| Teraspeed Labs Modeling Services.
| http://www.teraspeedlabs.com
[IBIS Ver]  4.0
[File Name] ev12ds400azpy-v2.ibs
[File Rev]  3.1
[Source]  Created by Teraspeed Labs LLC
[Date]   05/12/2015
[Notes]   Quality Check of this IBIS model: Model Passes IBIS Check
   Model parses into ICX IS. Simulation done with Hyperlynx.
   1. MIN TYP MAX information is based on Temperature and
   Voltage characteristics only.
   2. Package data gained using Tektronix IConnect Software.
   3. File Rev3.1: changed ball F10 from DGND to VCCD(from PDF)
[Disclaimer]
| Use: Teraspeed Labs  ("Teraspeed") has
| licensed IBIS models to specific integrated circuit
| suppliers ("IC Vendors") for use and distribution as
| follows: Each IC Vendor may use IBIS Models, and distribute
| them to IC Vendor's customers to use solely for developing
| printed circuit board designs. Users of this model may
| modify the IBIS model to suit its specific applications but
| rights to derivative works and such modifications shall belong
| to Teraspeed. No other distribution of these materials is
| permitted.
| DISCLAIMER OF WARRANTY: UNLESS OTHERWISE AGREED TO IN WRITING
| TERASPEED DISCLAIMS AND USER WAIVES ALL WARRANTIES, EXPRESS
| OR IMPLIED, INCLUDING WARRANTIES OF MERCHANTABILITY AND
| FITNESS FOR A PARTICULAR PURPOSE. IN NO EVENT SHALL
| TERASPEED BE LIABLE FOR ANY DIRECT OR INDIRECT DAMAGES,
| WHETHER IN CONTRACT OR TORT, INCLUDING, WITHOUT LIMITATION,
| LOST PROFITS, BUSINESS INTERRUPTION, OR LOST INFORMATION
| ARISING OUT OF THE USE OF OR THE INABILITY TO USE THE MODEL,
| EVEN IF TERASPEED HAS BEEN ADVISED OF THE POSSIBILITY OF SUCH
| DAMAGES.
[Copyright]
| This file is the legal property of Teraspeed Labs Copyright(c) 2015.
| All other rights are reserved.
[Component]   EV12DS400AZPY-v2
[Manufacturer] e2v semiconductors
| Data Sheet: Preliminary - SEPT 14/Extract of Product Brief
[Package]
| FpBGA196 ROHS
| variable   typ   min   max
R_pkg  1.000E-02   1.000E-02   1.000E-02
L_pkg  1.293E-09   1.711E-10   2.224E-09
C_pkg  4.897E-13   6.478E-14   8.421E-13
[Pin] signal_name   model_name   R_pin   L_pin   C_pin
A1   DGND   GND   1.000E-02   2.224E-09   8.421E-13
A2   B5   lvds_in   1.000E-02   2.060E-09   7.800E-13
A3   B6   lvds_in   1.000E-02   1.913E-09   7.242E-13
A4   B6N   lvds_in   1.000E-02   1.786E-09   6.763E-13
A5   B9   lvds_in   1.000E-02   1.685E-09   6.380E-13
A6   B9N   lvds_in   1.000E-02   1.614E-09   6.111E-13
A7   B11   lvds_in   1.000E-02   1.577E-09   5.972E-13
A8   C11   lvds_in   1.000E-02   1.577E-09   5.972E-13
A9   C9N   lvds_in   1.000E-02   1.614E-09   6.111E-13
A10   C9   lvds_in   1.000E-02   1.685E-09   6.380E-13
A11   C6N   lvds_in   1.000E-02   1.786E-09   6.763E-13
A12   C6   lvds_in   1.000E-02   1.913E-09   7.242E-13
A13   C5   lvds_in   1.000E-02   2.060E-09   7.800E-13
A14   DGND   GND   1.000E-02   2.224E-09   8.421E-13
B1   B3   lvds_in   1.000E-02   2.060E-09   7.800E-13
B2   B4   lvds_in   1.000E-02   1.882E-09   7.125E-13
B3   B5N   lvds_in   1.000E-02   1.719E-09   6.510E-13
B4   B7   lvds_in   1.000E-02   1.577E-09   5.972E-13
B5   B8   lvds_in   1.000E-02   1.462E-09   5.534E-13
B6   B10   lvds_in   1.000E-02   1.379E-09   5.222E-13
B7   B11N   lvds_in   1.000E-02   1.336E-09   5.059E-13
B8   C11N   lvds_in   1.000E-02   1.336E-09   5.059E-13
B9   C10   lvds_in   1.000E-02   1.379E-09   5.222E-13
B10   C8   lvds_in   1.000E-02   1.462E-09   5.534E-13
B11   C7   lvds_in   1.000E-02   1.577E-09   5.972E-13
B12   C5N   lvds_in   1.000E-02   1.719E-09   6.510E-13
B13   C4   lvds_in   1.000E-02   1.882E-09   7.125E-13
B14   C3   lvds_in   1.000E-02   2.060E-09   7.800E-13
C1   B1N   lvds_in   1.000E-02   1.913E-09   7.242E-13
C2   B3N   lvds_in   1.000E-02   1.719E-09   6.510E-13
C3   B4N   lvds_in   1.000E-02   1.540E-09   5.830E-13
C4   B7N   lvds_in   1.000E-02   1.379E-09   5.222E-13
C5   B8N   lvds_in   1.000E-02   1.245E-09   4.716E-13
C6   B10N   lvds_in   1.000E-02   1.148E-09   4.345E-13
C7   DGND   GND   1.000E-02   1.095E-09   4.148E-13
C8   DGND   GND   1.000E-02   1.095E-09   4.148E-13
C9   C10N   lvds_in   1.000E-02   1.148E-09   4.345E-13
C10   C8N   lvds_in   1.000E-02   1.245E-09   4.716E-13
C11   C7N   lvds_in   1.000E-02   1.379E-09   5.222E-13
C12   C4N   lvds_in   1.000E-02   1.540E-09   5.830E-13
C13   C3N   lvds_in   1.000E-02   1.719E-09   6.510E-13
C14   C1N   lvds_in   1.000E-02   1.913E-09   7.242E-13
D1   B1   lvds_in   1.000E-02   1.786E-09   6.763E-13
D2   B2   lvds_in   1.000E-02   1.577E-09   5.972E-13
D3   B2N   lvds_in   1.000E-02   1.379E-09   5.222E-13
D4   DGND   GND   1.000E-02   1.198E-09   4.534E-13
D5   DGND   GND   1.000E-02   1.041E-09   3.940E-13
D6   VCCD   POWER   1.000E-02   9.213E-10   3.488E-13
D7   VCCD   POWER   1.000E-02   8.554E-10   3.239E-13
D8   VCCD   POWER   1.000E-02   8.554E-10   3.239E-13
D9   VCCD   POWER   1.000E-02   9.213E-10   3.488E-13
D10   DGND   GND   1.000E-02   1.041E-09   3.940E-13
D11   DGND   GND   1.000E-02   1.198E-09   4.534E-13
D12   C2N   lvds_in   1.000E-02   1.379E-09   5.222E-13
D13   C2   lvds_in   1.000E-02   1.577E-09   5.972E-13
D14   C1   lvds_in   1.000E-02   1.786E-09   6.763E-13
E1   A10N   lvds_in   1.000E-02   1.685E-09   6.380E-13
E2   B0   lvds_in   1.000E-02   1.462E-09   5.534E-13
E3   B0N   lvds_in   1.000E-02   1.245E-09   4.716E-13
E4   DGND   GND   1.000E-02   1.041E-09   3.940E-13
E5   DGND   GND   1.000E-02   8.554E-10   3.239E-13
E6   VCCD   POWER   1.000E-02   7.054E-10   2.671E-13
E7   VCCD   POWER   1.000E-02   6.168E-10   2.336E-13
E8   VCCD   POWER   1.000E-02   6.168E-10   2.336E-13
E9   VCCD   POWER   1.000E-02   7.054E-10   2.671E-13
E10   DGND   GND   1.000E-02   8.554E-10   3.239E-13
E11   DGND   GND   1.000E-02   1.041E-09   3.940E-13
E12   C0N   lvds_in   1.000E-02   1.245E-09   4.716E-13
E13   C0   lvds_in   1.000E-02   1.462E-09   5.534E-13
E14   D10N   lvds_in   1.000E-02   1.685E-09   6.380E-13
F1   A10   lvds_in   1.000E-02   1.614E-09   6.111E-13
F2   A11   lvds_in   1.000E-02   1.379E-09   5.222E-13
F3   A11N   lvds_in   1.000E-02   1.148E-09   4.345E-13
F4   VCCD   POWER   1.000E-02   9.213E-10   3.488E-13
F5   VCCD   POWER   1.000E-02   7.054E-10   2.671E-13
F6   AGND   GND   1.000E-02   5.132E-10   1.943E-13
F7   AGND   GND   1.000E-02   3.825E-10   1.448E-13
F8   AGND   GND   1.000E-02   3.825E-10   1.448E-13
F9   AGND   GND   1.000E-02   5.132E-10   1.943E-13
F10   VCCD   POWER   1.000E-02   7.054E-10   2.671E-13
F11   VCCD   POWER   1.000E-02   9.213E-10   3.488E-13
F12   D11N   lvds_in   1.000E-02   1.148E-09   4.345E-13
F13   D11   lvds_in   1.000E-02   1.379E-09   5.222E-13
F14   D10   lvds_in   1.000E-02   1.614E-09   6.111E-13
G1   A8   lvds_in   1.000E-02   1.577E-09   5.972E-13
G2   A8N   lvds_in   1.000E-02   1.336E-09   5.059E-13
G3   A9   lvds_in   1.000E-02   1.095E-09   4.148E-13
G4   A9N   lvds_in   1.000E-02   8.554E-10   3.239E-13
G5   DGND   GND   1.000E-02   6.168E-10   2.336E-13
G6   AGND   GND   1.000E-02   3.825E-10   1.448E-13
G7   AGND   GND   1.000E-02   1.711E-10   6.478E-14
G8   AGND   GND   1.000E-02   1.711E-10   6.478E-14
G9   AGND   GND   1.000E-02   3.825E-10   1.448E-13
G10   DGND   GND   1.000E-02   6.168E-10   2.336E-13
G11   D9N   lvds_in   1.000E-02   8.554E-10   3.239E-13
G12   D9   lvds_in   1.000E-02   1.095E-09   4.148E-13
G13   D8N   lvds_in   1.000E-02   1.336E-09   5.059E-13
G14   D8   lvds_in   1.000E-02   1.577E-09   5.972E-13
H1   A6   lvds_in   1.000E-02   1.577E-09   5.972E-13
H2   A6N   lvds_in   1.000E-02   1.336E-09   5.059E-13
H3   A7   lvds_in   1.000E-02   1.095E-09   4.148E-13
H4   A7N   lvds_in   1.000E-02   8.554E-10   3.239E-13
H5   DGND   GND   1.000E-02   6.168E-10   2.336E-13
H6   AGND   GND   1.000E-02   3.825E-10   1.448E-13
H7   AGND   GND   1.000E-02   1.711E-10   6.478E-14
H8   AGND   GND   1.000E-02   1.711E-10   6.478E-14
H9   AGND   GND   1.000E-02   3.825E-10   1.448E-13
H10   DGND   GND   1.000E-02   6.168E-10   2.336E-13
H11   D7N   lvds_in   1.000E-02   8.554E-10   3.239E-13
H12   D7   lvds_in   1.000E-02   1.095E-09   4.148E-13
H13   D6N   lvds_in   1.000E-02   1.336E-09   5.059E-13
H14   D6   lvds_in   1.000E-02   1.577E-09   5.972E-13
J1   A3N   lvds_in   1.000E-02   1.614E-09   6.111E-13
J2   A5   lvds_in   1.000E-02   1.379E-09   5.222E-13
J3   A5N   lvds_in   1.000E-02   1.148E-09   4.345E-13
J4   VCCA3   POWER   1.000E-02   9.213E-10   3.488E-13
J5   VCCA3   POWER   1.000E-02   7.054E-10   2.671E-13
J6   AGND   GND   1.000E-02   5.132E-10   1.943E-13
J7   AGND   GND   1.000E-02   3.825E-10   1.448E-13
J8   AGND   GND   1.000E-02   3.825E-10   1.448E-13
J9   AGND   GND   1.000E-02   5.132E-10   1.943E-13
J10   VCCA3   POWER   1.000E-02   7.054E-10   2.671E-13
J11   VCCA3   POWER   1.000E-02   9.213E-10   3.488E-13
J12   D5N   lvds_in   1.000E-02   1.148E-09   4.345E-13
J13   D5   lvds_in   1.000E-02   1.379E-09   5.222E-13
J14   D3N   lvds_in   1.000E-02   1.614E-09   6.111E-13
K1   A3   lvds_in   1.000E-02   1.685E-09   6.380E-13
K2   A4   lvds_in   1.000E-02   1.462E-09   5.534E-13
K3   A4N   lvds_in   1.000E-02   1.245E-09   4.716E-13
K4   DGND   GND   1.000E-02   1.041E-09   3.940E-13
K5   DGND   GND   1.000E-02   8.554E-10   3.239E-13
K6   AGND   GND   1.000E-02   7.054E-10   2.671E-13
K7   VCCA5   POWER   1.000E-02   6.168E-10   2.336E-13
K8   VCCA5   POWER   1.000E-02   6.168E-10   2.336E-13
K9   AGND   GND   1.000E-02   7.054E-10   2.671E-13
K10   DGND   GND   1.000E-02   8.554E-10   3.239E-13
K11   DGND   GND   1.000E-02   1.041E-09   3.940E-13
K12   D4N   lvds_in   1.000E-02   1.245E-09   4.716E-13
K13   D4   lvds_in   1.000E-02   1.462E-09   5.534E-13
K14   D3   lvds_in   1.000E-02   1.685E-09   6.380E-13
L1   A1N   lvds_in   1.000E-02   1.786E-09   6.763E-13
L2   A2   lvds_in   1.000E-02   1.577E-09   5.972E-13
L3   A2N   lvds_in   1.000E-02   1.379E-09   5.222E-13
L4   DGND   GND   1.000E-02   1.198E-09   4.534E-13
L5   DIODE   term   1.000E-02   1.041E-09   3.940E-13
L6   VCCA5   POWER   1.000E-02   9.213E-10   3.488E-13
L7   VCCA5   POWER   1.000E-02   8.554E-10   3.239E-13
L8   VCCA5   POWER   1.000E-02   8.554E-10   3.239E-13
L9   VCCA5   POWER   1.000E-02   9.213E-10   3.488E-13
L10   DGND   GND   1.000E-02   1.041E-09   3.940E-13
L11   SLD_N   spi_in   1.000E-02   1.198E-09   4.534E-13
L12   D2N   lvds_in   1.000E-02   1.379E-09   5.222E-13
L13   D2   lvds_in   1.000E-02   1.577E-09   5.972E-13
L14   D1N   lvds_in   1.000E-02   1.786E-09   6.763E-13
M1   A1   lvds_in   1.000E-02   1.913E-09   7.242E-13
M2   A0N   lvds_in   1.000E-02   1.719E-09   6.510E-13
M3   NC   NC   1.000E-02   1.540E-09   5.830E-13
|M4   TVF   cmos_out   1.000E-02   1.379E-09   5.222E-13
M5   RESET_N   spi_in   1.000E-02   1.245E-09   4.716E-13
M6   VCCA5   POWER   1.000E-02   1.148E-09   4.345E-13
M7   VCCA5   POWER   1.000E-02   1.095E-09   4.148E-13
M8   AGND   GND   1.000E-02   1.095E-09   4.148E-13
M9   AGND   GND   1.000E-02   1.148E-09   4.345E-13
M10   SDATA   spi_in   1.000E-02   1.245E-09   4.716E-13
M11   SCLK   spi_in   1.000E-02   1.379E-09   5.222E-13
M12   PSS2   ocds_pssx   1.000E-02   1.540E-09   5.830E-13
M13   D0N   lvds_in   1.000E-02   1.719E-09   6.510E-13
M14   D1   lvds_in   1.000E-02   1.913E-09   7.242E-13
N1   A0   lvds_in   1.000E-02   2.060E-09   7.800E-13
N2   DSPN   lvds_out   1.000E-02   1.882E-09   7.125E-13
N3   IDC_P   lvds_in   1.000E-02   1.719E-09   6.510E-13
N4   SYNCN   sync_in   1.000E-02   1.577E-09   5.972E-13
N5   CLKN   clk_in   1.000E-02   1.462E-09   5.534E-13
N6   AGND   GND   1.000E-02   1.379E-09   5.222E-13
N7   AGND   GND   1.000E-02   1.336E-09   5.059E-13
N8   AGND   GND   1.000E-02   1.336E-09   5.059E-13
N9   AGND   GND   1.000E-02   1.379E-09   5.222E-13
N10   AGND   GND   1.000E-02   1.462E-09   5.534E-13
N11   AGND   GND   1.000E-02   1.577E-09   5.972E-13
N12   IREF_TEST   NC   1.000E-02   1.719E-09   6.510E-13
N13   OCDS   ocds_pssx   1.000E-02   1.882E-09   7.125E-13
N14   D0   lvds_in   1.000E-02   2.060E-09   7.800E-13
P1   DGND   GND   1.000E-02   2.224E-09   8.421E-13
P2   DSP   lvds_out   1.000E-02   2.060E-09   7.800E-13
P3   IDC_N   lvds_in   1.000E-02   1.913E-09   7.242E-13
P4   SYNC   sync_in   1.000E-02   1.786E-09   6.763E-13
P5   CLK   clk_in   1.000E-02   1.685E-09   6.380E-13
P6   AGND   GND   1.000E-02   1.614E-09   6.111E-13
P7   AGND   GND   1.000E-02   1.577E-09   5.972E-13
P8   AGND   GND   1.000E-02   1.577E-09   5.972E-13
P9   OUT   term   1.000E-02   1.614E-09   6.111E-13
P10   OUTN   term   1.000E-02   1.685E-09   6.380E-13
P11   AGND   GND   1.000E-02   1.786E-09   6.763E-13
P12   PSS0   ocds_pssx   1.000E-02   1.913E-09   7.242E-13
P13   PSS1   ocds_pssx   1.000E-02   2.060E-09   7.800E-13
P14   DGND   GND   1.000E-02   2.224E-09   8.421E-13
[Diff Pin] inv_pin vdiff tdelay_typ tdelay_min tdelay_max
P5   N5   300mV   NA   NA   NA
N1   M2   100mV   NA   NA   NA
M1   L1   100mV   NA   NA   NA
F1   E1   100mV   NA   NA   NA
F2   F3   100mV   NA   NA   NA
L2   L3   100mV   NA   NA   NA
K1   J1   100mV   NA   NA   NA
K2   K3   100mV   NA   NA   NA
J2   J3   100mV   NA   NA   NA
H1   H2   100mV   NA   NA   NA
H3   H4   100mV   NA   NA   NA
G1   G2   100mV   NA   NA   NA
G3   G4   100mV   NA   NA   NA
E2   E3   100mV   NA   NA   NA
D1   C1   100mV   NA   NA   NA
B6   C6   100mV   NA   NA   NA
A7   B7   100mV   NA   NA   NA
D2   D3   100mV   NA   NA   NA
B1   C2   100mV   NA   NA   NA
B2   C3   100mV   NA   NA   NA
A2   B3   100mV   NA   NA   NA
A3   A4   100mV   NA   NA   NA
B4   C4   100mV   NA   NA   NA
B5   C5   100mV   NA   NA   NA
A5   A6   100mV   NA   NA   NA
E13   E12   100mV   NA   NA   NA
D14   C14   100mV   NA   NA   NA
B9   C9   100mV   NA   NA   NA
A10   A9   100mV   NA   NA   NA
A8   B8   100mV   NA   NA   NA
D13   D12   100mV   NA   NA   NA
B14   C13   100mV   NA   NA   NA
B13   C12   100mV   NA   NA   NA
A13   B12   100mV   NA   NA   NA
A12   A11   100mV   NA   NA   NA
B11   C11   100mV   NA   NA   NA
B10   C10   100mV   NA   NA   NA
M14   L14   100mV   NA   NA   NA
F14   E14   100mV   NA   NA   NA
G14   G13   100mV   NA   NA   NA
G12   G11   100mV   NA   NA   NA
F13   F12   100mV   NA   NA   NA
N14   M13   100mV   NA   NA   NA
L13   L12   100mV   NA   NA   NA
K14   J14   100mV   NA   NA   NA
K13   K12   100mV   NA   NA   NA
J13   J12   100mV   NA   NA   NA
H14   H13   100mV   NA   NA   NA
H12   H11   100mV   NA   NA   NA
N3   P3   100mV   NA   NA   NA
P4   N4   100mV   NA   NA   NA
P2   N2   NA   NA   NA   NA
[Series Pin Mapping] pin_2 model_name function_table_group
P5   N5   100ohm
N1   M2   100ohm
M1   L1   100ohm
F1   E1   100ohm
F2   F3   100ohm
L2   L3   100ohm
K1   J1   100ohm
K2   K3   100ohm
J2   J3   100ohm
H1   H2   100ohm
H3   H4   100ohm
G1   G2   100ohm
G3   G4   100ohm
E2   E3   100ohm
D1   C1   100ohm
B6   C6   100ohm
A7   B7   100ohm
D2   D3   100ohm
B1   C2   100ohm
B2   C3   100ohm
A2   B3   100ohm
A3   A4   100ohm
B4   C4   100ohm
B5   C5   100ohm
A5   A6   100ohm
E13   E12   100ohm
D14   C14   100ohm
B9   A9   100ohm
A10   C9   100ohm
A8   B8   100ohm
D13   D12   100ohm
B14   C13   100ohm
B13   C12   100ohm
A13   B12   100ohm
A12   A11   100ohm
B11   C11   100ohm
B10   C10   100ohm
M14   L14   100ohm
F14   G13   100ohm
G14   F12   100ohm
G12   G11   100ohm
F13   E14   100ohm
N14   M13   100ohm
L13   L12   100ohm
K14   J14   100ohm
K13   K12   100ohm
J13   J12   100ohm
H14   H13   100ohm
H12   H11   100ohm
N3   P3   100ohm
P4   N4   100ohm
[Model] 100ohm
Model_type  Series
C_comp   0  0  0
[Voltage Range]  3.3   3.15   3.45
[Temperature Range]  25   110   -40
[R series]   100   80   120
[Model] term
Model_type Terminator
C_comp   0  0  0
| variable   typ   min   max
[Voltage Range]   5.00V   4.75V   5.25V
[POWER Clamp Reference]  5.00V   4.75V   5.25V
[GND Clamp Reference]   0.00V   0.00V   0.00V
[Temperature Range]  25   110   -40
| Models and submodels in the file (8): clk_in (Input), lvds_in (Input), ocds_pssx (Input), spi_in (Input), sync_in (Input), lvds_out (Output), 100ohm (Series), term (Terminator)
